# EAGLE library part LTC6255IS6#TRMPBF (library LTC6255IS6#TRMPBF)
Precision Amplifiers Single 6.5MHz, 65uA, 1.8V to 5.25V, RRIO Op Amps Source: Datasheet
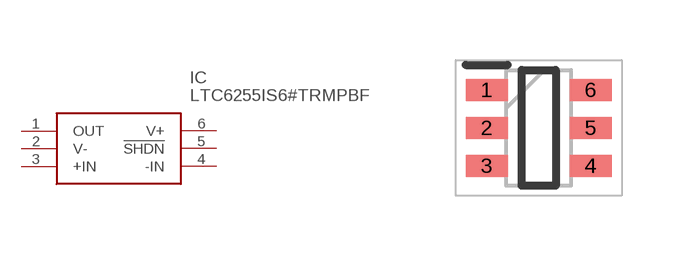
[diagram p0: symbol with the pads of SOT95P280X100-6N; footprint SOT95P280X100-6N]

Designator prefix IC

## LTC6255IS6#TRMPBF (Description: Precision Amplifiers Single 6.5MHz, 65uA, 1.8V to 5.25V, RRIO Op Amps; Height: 1mm; Manufacturer_Name: Analog Devices; Manufacturer_Part_Number: LTC6255IS6#TRMPBF; Mouser_Part_Number: 584-LTC6255IS6TRMPBF; Mouser_Price-Stock: https://www.mouser.co.uk/ProductDetail/Analog-Devices/LTC6255IS6TRMPBF?qs=hVkxg5c3xu%252BM0aXXLk0hVA%3D%3D)  [SOT95P280X100-6N]
1  OUT
2  V-
3  +IN
4  -IN
5  !SHDN
6  V+

## Footprint SOT95P280X100-6N (pad centres in mm)
6-Lead Plastic TSOT-23-1
smd 1.05 x 0.55: 1 -1.3,0.95; 2 -1.3,0; 3 -1.3,-0.95; 4 1.3,-0.95; 5 1.3,0; 6 1.3,0.95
